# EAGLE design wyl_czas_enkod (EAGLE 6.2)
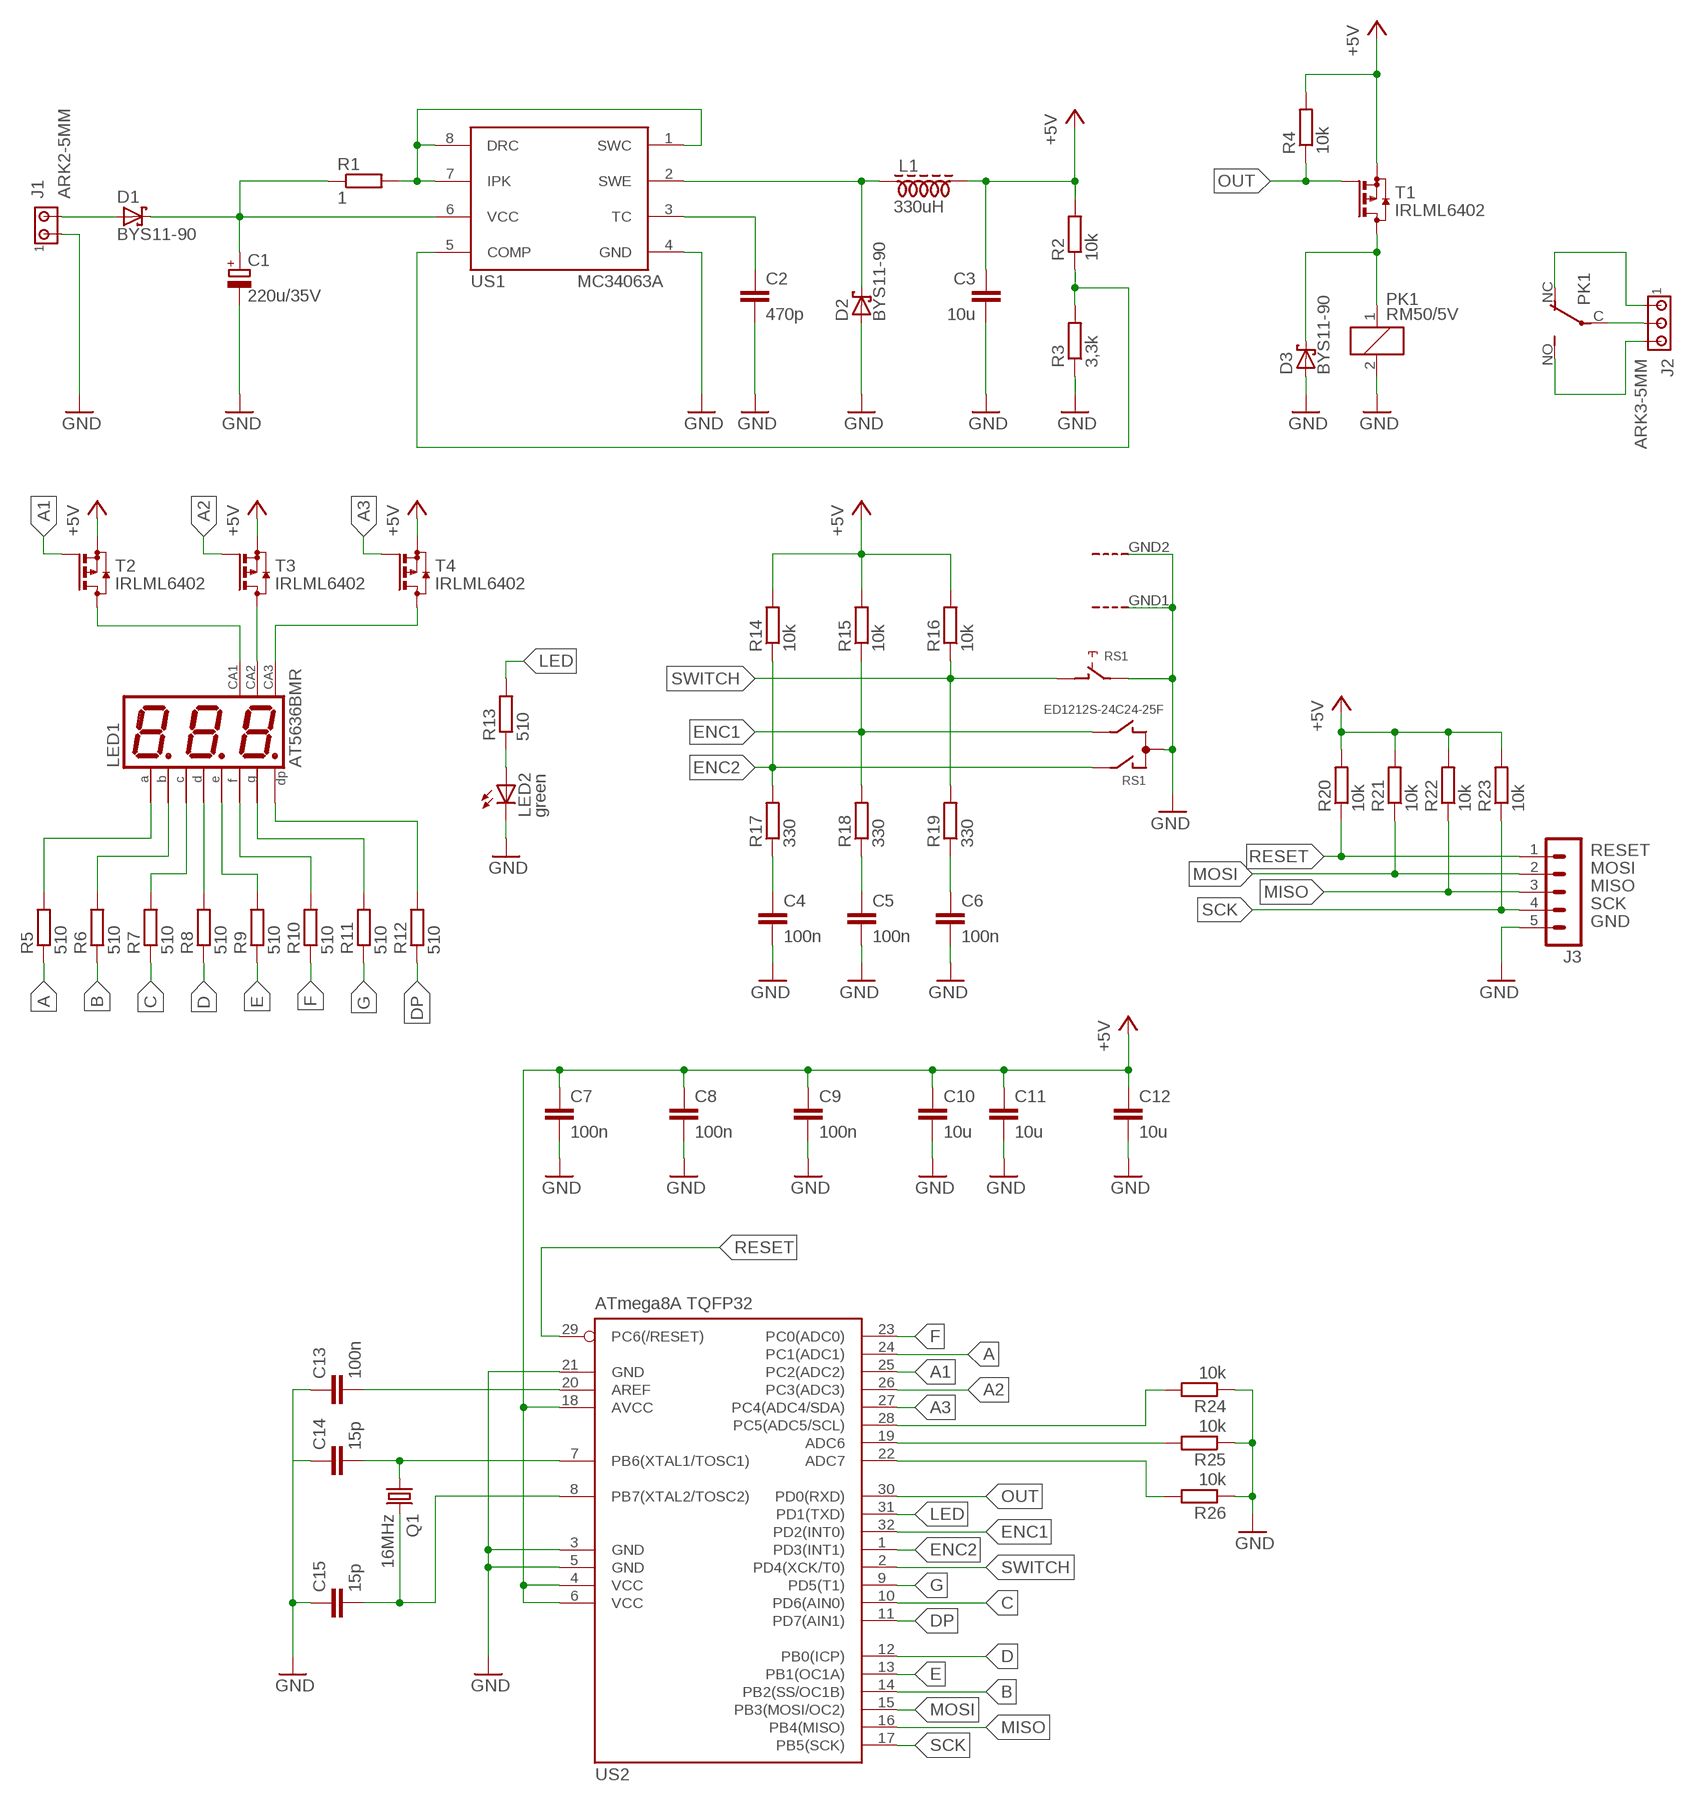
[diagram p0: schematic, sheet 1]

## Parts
C1  220u/35V  CPOL-EUE3.5-8  [E3,5-8]
C2  470p  C-EUC0805  [C0805]
C3  10u  C-EUC0805  [C0805]
C4  100n  C-EUC0805  [C0805]
C5  100n  C-EUC0805  [C0805]
C6  100n  C-EUC0805  [C0805]
C7  100n  C-EUC0805  [C0805]
C8  100n  C-EUC0805  [C0805]
C9  100n  C-EUC0805  [C0805]
C10  10u  C-EUC0805  [C0805]
C11  10u  C-EUC0805  [C0805]
C12  10u  C-EUC0805  [C0805]
C13  100n  C-EUC0805  [C0805]
C14  15p  C-EUC0805  [C0805]
C15  15p  C-EUC0805  [C0805]
D1  BYS11-90  SCHOTTKY-DIODESMD  [SMB]
D2  BYS11-90  SCHOTTKY-DIODESMD  [SMB]
D3  BYS11-90  SCHOTTKY-DIODESMD  [SMB]
J1  ARK2-5MM  [2PIN-5MM]
J2  ARK3-5MM  [3PIN-5MM]
J3  MA05-1  [MA05-1]
L1  330uH  DLAWIK-PION  [L_PION]
LED1  AT5636BMR  BC56-12SRWA  [BX56-12]
LED2  green  LED5MM  [LED5MM]
PK1  RM50/5V  PK_POJED-JQC-3FG  [PK_POJED_JQC-3FG]
Q1  16MHz  CRYSTALHC49UP  [HC49UP]
R1  1  R-EU_M0805  [M0805]
R2  10k  R-EU_M0805  [M0805]
R3  3,3k  R-EU_M0805  [M0805]
R4  10k  R-EU_M0805  [M0805]
R5  510  R-EU_M0805  [M0805]
R6  510  R-EU_M0805  [M0805]
R7  510  R-EU_M0805  [M0805]
R8  510  R-EU_M0805  [M0805]
R9  510  R-EU_M0805  [M0805]
R10  510  R-EU_M0805  [M0805]
R11  510  R-EU_M0805  [M0805]
R12  510  R-EU_M0805  [M0805]
R13  510  R-EU_M0805  [M0805]
R14  10k  R-EU_R0805  [R0805]
R15  10k  R-EU_R0805  [R0805]
R16  10k  R-EU_R0805  [R0805]
R17  330  R-EU_R0805  [R0805]
R18  330  R-EU_R0805  [R0805]
R19  330  R-EU_R0805  [R0805]
R20  10k  R-EU_R0805  [R0805]
R21  10k  R-EU_R0805  [R0805]
R22  10k  R-EU_R0805  [R0805]
R23  10k  R-EU_R0805  [R0805]
R24  10k  R-EU_R0805  [R0805]
R25  10k  R-EU_R0805  [R0805]
R26  10k  R-EU_R0805  [R0805]
RS1  ED1212S-24C24-25F  EC12E_SW  [ALPS_EC12E_SW]
T1  IRLML6402  BSS84  [SOT23]
T2  IRLML6402  BSS84  [SOT23]
T3  IRLML6402  BSS84  [SOT23]
T4  IRLML6402  BSS84  [SOT23]
US1  MC34063A  MC34063-SO8  [SO08]
US2  ATmega8A TQFP32  MEGA8-AI  [TQFP32-08]

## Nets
+5V: C3.1 C7.1 C8.1 C9.1 C10.1 C11.1 C12.1 L1.P$2 R2.2 R4.2 R14.2 R15.2 R16.2 R20.2 R21.2 R22.2 R23.2 T1.2(S) T2.2(S) T3.2(S) T4.2(S) US2.4(VCC) US2.6(VCC) US2.18(AVCC)
A: R5.1 US2.24(PC1(ADC1))
A1: T2.1(G) US2.25(PC2(ADC2))
A2: T3.1(G) US2.26(PC3(ADC3))
A3: T4.1(G) US2.27(PC4(ADC4/SDA))
B: R6.1 US2.14(PB2(SS/OC1B))
C: R7.1 US2.10(PD6(AIN0))
D: R8.1 US2.12(PB0(ICP))
DP: R12.1 US2.11(PD7(AIN1))
E: R9.1 US2.13(PB1(OC1A))
ENC1: R15.1 R18.2 RS1.B US2.32(PD2(INT0))
ENC2: R14.1 R17.2 RS1.A US2.1(PD3(INT1))
F: R10.1 US2.23(PC0(ADC0))
G: R11.1 US2.9(PD5(T1))
GND: C1.- C2.2 C3.2 C4.2 C5.2 C6.2 C7.2 C8.2 C9.2 C10.2 C11.2 C12.2 C13.1 C14.1 C15.1 D2.A D3.A J1.P$1 J3.5 LED2.K(C) PK1.2 R3.1 R24.1 R25.1 R26.1 RS1.C RS1.E RS1.GND1(G) RS1.GND2(G) US1.4(GND) US2.3(GND) US2.5(GND) US2.21(GND)
LED: R13.2 US2.31(PD1(TXD))
MISO: J3.3 R22.1 US2.16(PB4(MISO))
MOSI: J3.2 R21.1 US2.15(PB3(MOSI/OC2))
N$1: C6.1 R19.1
N$2: LED2.A R13.1
N$3: C15.2 Q1.2 US2.8(PB7(XTAL2/TOSC2))
N$4: C13.2 US2.20(AREF)
N$5: R25.2 US2.19(ADC6)
N$6: R24.2 US2.28(PC5(ADC5/SCL))
N$7: J2.P$1 PK1.NC
N$8: J2.P$3 PK1.NO
N$9: R2.1 R3.2 US1.5(COMP)
N$10: C14.2 Q1.1 US2.7(PB6(XTAL1/TOSC1))
N$11: LED1.9(CA) T3.3(D)
N$12: R26.2 US2.22(ADC7)
N$14: LED1.12(CA) T2.3(D)
N$15: LED1.8(CA) T4.3(D)
N$16: LED1.11(A) R5.2
N$17: LED1.7(B) R6.2
N$18: LED1.4(C) R7.2
N$19: LED1.2(D) R8.2
N$20: LED1.1(E) R9.2
N$21: LED1.10(F) R10.2
N$22: LED1.5(G) R11.2
N$23: LED1.3(DP) R12.2
N$31: D1.A J1.P$2
N$32: C1.+ D1.C R1.1 US1.6(VCC)
N$34: J2.P$2 PK1.C(COM)
N$35: C5.1 R18.1
N$36: C4.1 R17.1
N$37: R1.2 US1.1(SWC) US1.7(IPK) US1.8(DRC)
N$38: C2.1 US1.3(TC)
N$39: D2.C L1.P$1 US1.2(SWE)
N$40: D3.C PK1.1 T1.3(D)
OUT: R4.1 T1.1(G) US2.30(PD0(RXD))
RESET: J3.1 R20.1 US2.29(PC6(/RESET))
SCK: J3.4 R23.1 US2.17(PB5(SCK))
SWITCH: R16.1 R19.2 RS1.D US2.2(PD4(XCK/T0))

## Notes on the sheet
- RESET
- MOSI
- MISO
- SCK
- GND

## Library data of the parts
C1 = rcl:CPOL-EU: POLARIZED CAPACITOR, European symbol
C2-C15 = rcl:C-EU: CAPACITOR, European symbol
D1-D3 = diode:SCHOTTKY-DIODE: Schottky Diode
J1 = zlacza_futrzak:ARK2: ARK 2
J2 = zlacza_futrzak:ARK3: ARK 3 Raster 5mm i 3,5mm
J3 = zlacza_futrzak:MA05-1: PIN HEADER; OC_FARNELL: unknown; OC_NEWARK: unknown
L1 = inne_futrzak:DLAWIK
LED1 = display-kingbright:B?56-12*WA: 14.22mm (0.56INCH) THREE DIGIT NUMERIC DISPLAY Source: http://www.kingbright.com .. BA56-11EWA(Ver1189474895.pdf; OC_FARNELL: unknown; OC_NEWARK: unknown
LED2 = led:LED: LED
PK1 = inne_futrzak:PK_POJED
Q1 = crystal:CRYSTAL: CRYSTAL; OC_FARNELL: unknown; OC_NEWARK: unknown
R1-R26 = rcl:R-EU_: RESISTOR, European symbol
RS1 = switch-alps:EC12E_SW: ALPS rotary Encoder EC12E series with switch; MPN: EC12E2424407; OC_FARNELL: 1520813; OC_NEWARK: 74M1068
T1-T4 = transistor-small-signal:BSS84: P-CHANNEL MOS FET
US1 = scalaki_futrzak:MC34063
US2 = atmel:MEGA8: MICROCONTROLLER 8 Kbytes FLASH, 1 kbytes SRAM, 512 bytes EEPROM, USART, 6-channel 10 bit ADC, 2-channel 8 bit ADC Pin compatible with Atmega48, ATMega88, ATMega168 Source: avr.lbr; MPN: ATMEGA8-16AU; OC_FARNELL: 9171371; OC_NEWARK: 73M8863

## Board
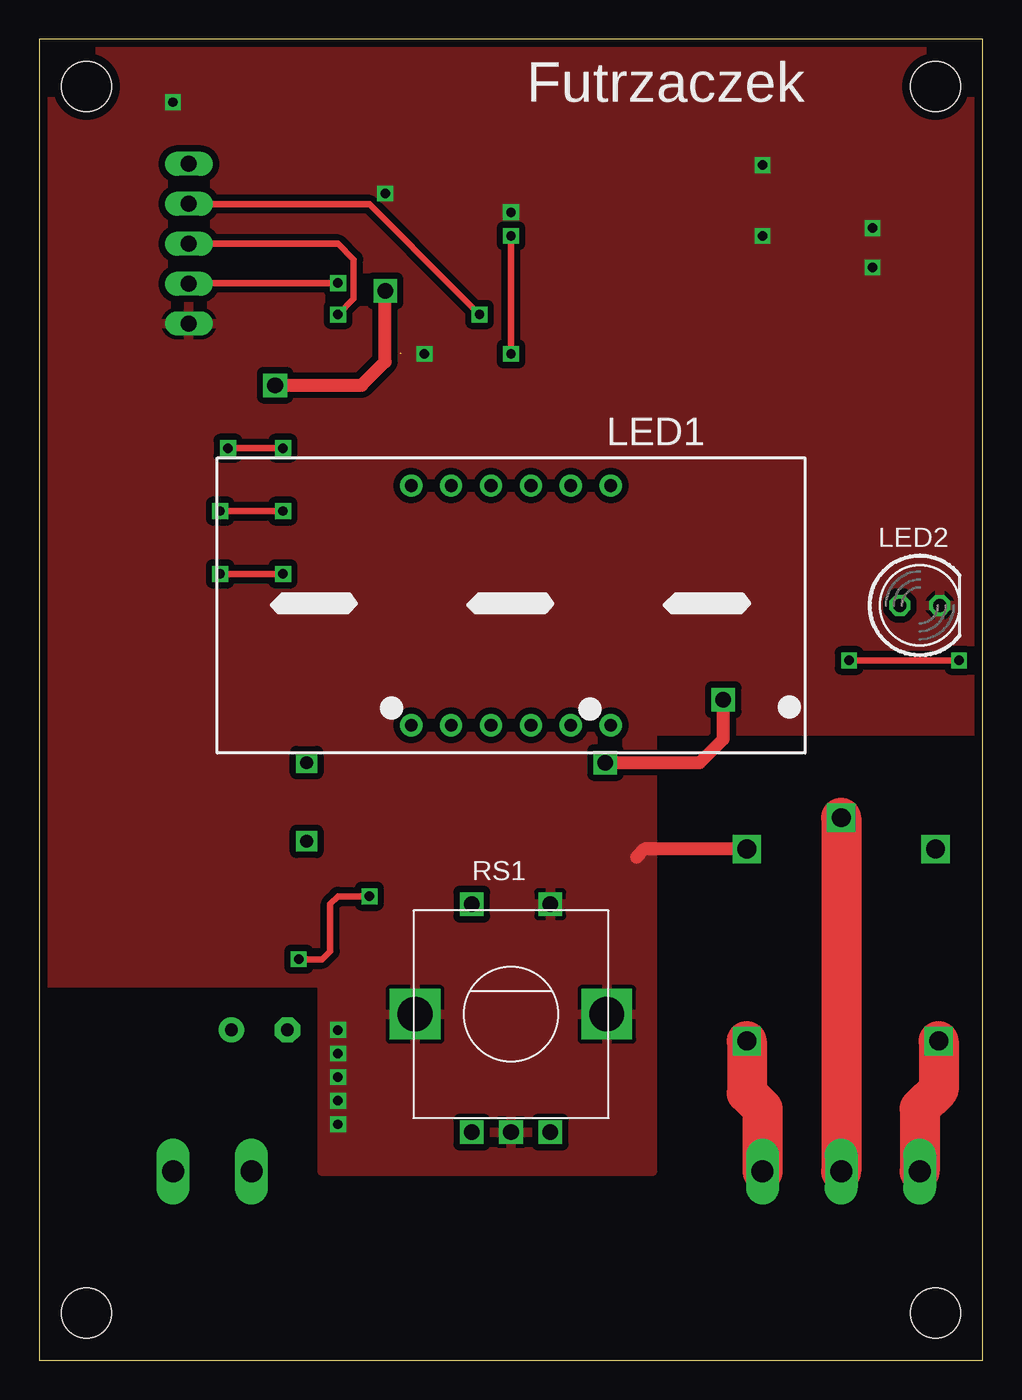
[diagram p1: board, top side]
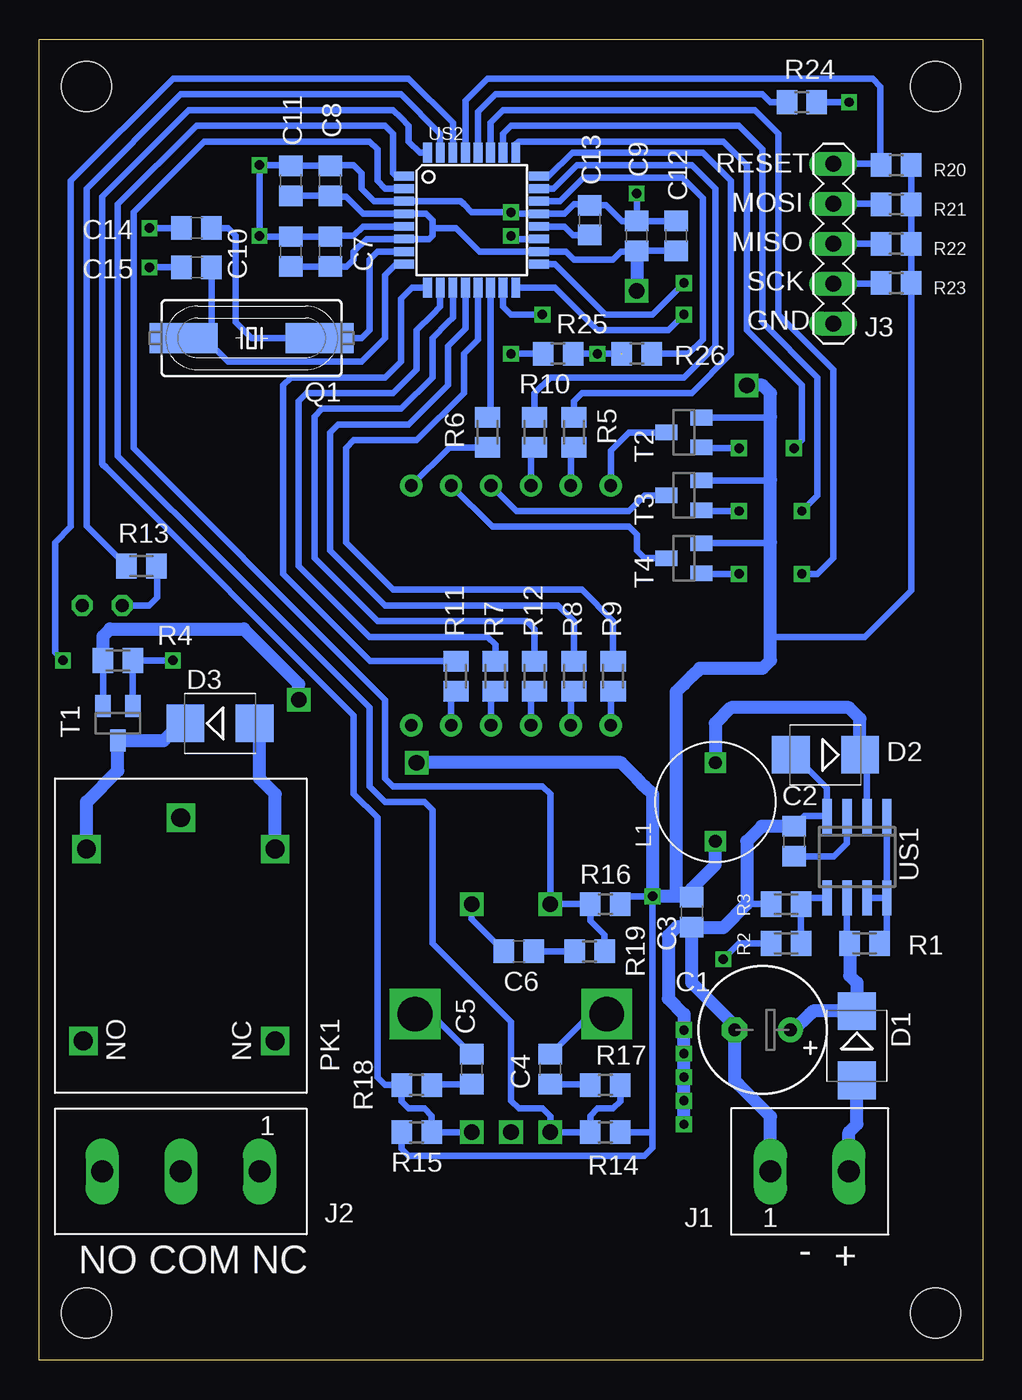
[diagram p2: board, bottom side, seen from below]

Size 60 x 84 mm. Coordinates in mm from the lower left corner, seen from the top.
Outline: 0,0 60,0 60,84 0,84 0,0
Copper layers (1*16): Top 0.035mm / dielectric 1.5mm / Bottom 0.035mm
Design rules: minimum track width 10mil, minimum drill 23mil, track to track 8mil, track to pad 8mil, pad to pad 8mil, via to via 8mil, smd to smd 8mil, copper to edge 20mil, drill to drill 8mil, minimum pad ring 10mil, minimum via ring 8mil, stop-mask expansion 4mil, vias tented up to drill 0mil, thermal gap 10mil
Holes 3.2 mm at 3,3 57,3 3,81 57,81

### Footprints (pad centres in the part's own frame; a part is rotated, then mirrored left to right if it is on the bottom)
E3,5-8 = drill 0.813 pad 1.6: + -1.778,0 | drill 0.813 pad 1.6 octagon: - 1.778,0
C0805 = smd 1.3 x 1.5: 1 -0.95,0; 2 0.95,0
SMB = smd 2.4 x 2.4: A 2.2,0; C -2.2,0
2PIN-5MM = drill 1.4 long: P$1 -2.5,0; P$2 2.5,0
3PIN-5MM = drill 1.4 long: P$1 -5,0; P$2 0,0; P$3 5,0
MA05-1 = drill 1.016 long: 1 -5.08,0; 2 -2.54,0; 3 0,0; 4 2.54,0; 5 5.08,0
L_PION = drill 0.8 square: P$1 -2.5,0; P$2 2.5,0
BX56-12 = drill 0.8 pad 1.422: 1 -6.35,-7.62; 2 -3.81,-7.62; 3 -1.27,-7.62; 4 1.27,-7.62; 5 3.81,-7.62; 6 6.35,-7.62; 7 6.35,7.62; 8 3.81,7.62; 9 1.27,7.62; 10 -1.27,7.62; 11 -3.81,7.62; 12 -6.35,7.62
LED5MM = drill 0.813 octagon: A -1.27,0; K 1.27,0
PK_POJED_JQC-3FG = drill 1.2 square: 1 5.5,6; 2 5.5,-6; C 7.5,0; NC -6.7,-6; NO -6.7,6.2
HC49UP = smd 4.318 x 1.93: 1 -4.318,0; 2 4.318,0
M0805 = smd 1.3 x 1.6: 1 -0.95,0; 2 0.95,0
R0805 = smd 1.3 x 1.5: 1 -0.95,0; 2 0.95,0
ALPS_EC12E_SW = drill 1 square: A -2.5,-7.5; B 2.5,-7.5; C 0,-7.5; D -2.5,7; E 2.5,7 | drill 2.2 square: GND1 -6.1,0; GND2 6.1,0
SOT23 = smd 1 x 1.4: 1 -0.95,-1.1; 2 0.95,-1.1; 3 0,1.1
SO08 = smd 0.6 x 2.2: 1 -1.905,-2.6; 2 -0.635,-2.6; 3 0.635,-2.6; 4 1.905,-2.6; 5 1.905,2.6; 6 0.635,2.6; 7 -0.635,2.6; 8 -1.905,2.6
TQFP32-08 = smd 1.27 x 0.559: 1 -4.293,2.8; 2 -4.293,2; 3 -4.293,1.2; 4 -4.293,0.4; 5 -4.293,-0.4; 6 -4.293,-1.2; 7 -4.293,-2; 8 -4.293,-2.8; 17 4.293,-2.8; 18 4.293,-2; 19 4.293,-1.2; 20 4.293,-0.4; 21 4.293,0.4; 22 4.293,1.2; 23 4.293,2; 24 4.293,2.8 | smd 0.559 x 1.27: 9 -2.8,-4.293; 10 -2,-4.293; 11 -1.2,-4.293; 12 -0.4,-4.293; 13 0.4,-4.293; 14 1.2,-4.293; 15 2,-4.293; 16 2.8,-4.293; 25 2.8,4.293; 26 2,4.293; 27 1.2,4.293; 28 0.4,4.293; 29 -0.4,4.293; 30 -1.2,4.293; 31 -2,4.293; 32 -2.8,4.293

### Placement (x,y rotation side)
C1  14,21 180 bottom
C2  12,33 90 bottom
C3  18.5,28.5 270 bottom
C4  27.5,18.5 90 bottom
C5  32.5,18.5 90 bottom
C6  29.5,26 180 bottom
C7  41.5,70.5 90 bottom
C8  41.5,75 90 bottom
C9  22,71.5 90 bottom
C10  44,70.5 90 bottom
C11  44,75 90 bottom
C12  19.5,71.5 90 bottom
C13  25,72.5 270 bottom
C14  50,72 0 bottom
C15  50,69.5 0 bottom
D1  8,20 270 bottom
D2  10,38.5 180 bottom
D3  48.5,40.5 0 bottom
J1  11,12 0 bottom
J2  51,12 180 bottom
J3  9.5,71 270 bottom
L1  17,35.5 270 bottom
LED1  30,48 0 top
LED2  56,48 0 top
PK1  51,27 90 bottom
Q1  46.5,65 180 bottom
R1  7.5,26.5 0 bottom
R2  12.5,26.5 180 bottom
R3  12.5,29 0 bottom
R4  55,44.5 180 bottom
R5  26,59 270 bottom
R6  31.5,59 270 bottom
R7  31,43.5 270 bottom
R8  26,43.5 270 bottom
R9  23.5,43.5 270 bottom
R10  28.5,59 270 bottom
R11  33.5,43.5 270 bottom
R12  28.5,43.5 270 bottom
R13  53.5,50.5 180 bottom
R14  24,14.5 0 bottom
R15  36,14.5 180 bottom
R16  24,29 0 bottom
R17  24,17.5 0 bottom
R18  36,17.5 180 bottom
R19  25,26 0 bottom
R20  5.5,76 0 bottom
R21  5.5,73.5 0 bottom
R22  5.5,71 0 bottom
R23  5.5,68.5 0 bottom
R24  11.5,80 180 bottom
R25  27,64 180 bottom
R26  22,64 0 bottom
RS1  30,22 0 top
T1  55,40.5 180 bottom
T2  19,59 90 bottom
T3  19,55 90 bottom
T4  19,51 90 bottom
US1  8,32 180 bottom
US2  32.5,72.5 0 bottom

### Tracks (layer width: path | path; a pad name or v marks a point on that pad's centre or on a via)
+5V  (via drill 0.6, 1)
  Top 0.406: v16.5,25.5 18,25.5 18.5,26 18.5,29 19,29.5 v21,29.5
  Top 0.813: v36,38 42,38 43.5,39.5 v43.5,42 | v15,62 19,62 20.5,62 22,63.5 v22,68
  Bottom 0.406: R2.2 15.5,26.5 16,26 v16.5,25.5 | 18.55,29.5 C3.1 | R15.2 36.95,13.45 36.5,13 21.5,13 21,13.5 21,14.5 | 21,14.5 v21,29.5 22.5,29.5 23,29 R16.2 | R14.2 21,14.5 | R4.2 T1.2 | T4.2 13.55,51.95 13.5,52 | T2.2 13.55,59.95 13.5,60 | T3.2 13.55,55.95 13.5,56 | C12.1 C9.1 22.05,70.5 23,70.5 23.5,70 26,70 26.5,70.5 US2.18 30.5,70.5 32,70.5 33.5,72 35,72 | C11.1 C8.1 41.45,74 40.5,74 39.4,72.9 US2.4 35.4,72.9 35,72.5 35,72 | C10.1 C7.1 40.45,69.55 40,70 40,70.5 39.2,71.3 US2.6 35.2,71.3 35,71.5 35,72 | R20.2 R21.2 R22.2 R23.2 4.55,48.95 7.5,46 13.5,46
  Bottom 0.813: C3.1 18.5,30 17,31.5 L1.P$2 | R4.2 55.95,46.05 55.5,46.5 47,46.5 43.5,43 v43.5,42 | 18.55,29.5 19.5,29.5 | 19.5,29.5 v21,29.5 21,36 21.5,36.5 22,37 23,38 v36,38 | 19.5,29.5 19.5,42.5 19,43 18.5,43.5 18,44 14,44 13.5,44.5 13.5,46 13.5,52 13.5,56 13.5,60 13.5,61.5 14,62 v15,62 | C9.1 v22,68
A
  Bottom 0.406: R5.1 26,61 25.5,61.5 24.45,61.5 18.5,61.5 16,64 16,75 16.5,75.5 17.5,76.5 17.8,76.8 26.1,76.8 27.6,75.3 US2.24
A1  (via drill 0.6)
  Top 0.406: v12,58 v15.5,58
  Bottom 0.406: US2.25 29.7,77.3 29.5,77.5 16.5,77.5 15.5,76.5 15,76 15,65.5 11.5,62 11.5,58.5 v12,58 | v15.5,58 17.85,58 T2.1
A2  (via drill 0.6)
  Top 0.406: v11.5,54 v15.5,54
  Bottom 0.406: US2.26 30.5,78 30,78.5 15.5,78.5 14.5,77.5 14,77 14,66 10.5,62.5 10.5,55 v11.5,54 | v15.5,54 17.85,54 T3.1
A3  (via drill 0.6)
  Top 0.406: v11.5,50 v15.5,50
  Bottom 0.406: US2.27 31.3,78.7 30.5,79.5 14.5,79.5 13.5,78.5 13,78 13,66.5 9.5,63 9.5,51 10.5,50 v11.5,50 | v15.5,50 17.85,50 T4.1
B
  Bottom 0.406: US2.14 31.3,60.15 R6.1
C
  Bottom 0.406: R7.1 31,45.5 31.5,46 39,46 43.5,50.5 43.5,61 43,61.5 37.5,61.5 36,63 36,65.5 35,66.5 34.5,67 US2.10
D
  Bottom 0.406: R8.1 26,47 27,48 38,48 41.5,51.5 41.5,59 41,59.5 36.5,59.5 34,62 34,64.5 33,65.5 32.9,65.6 US2.12
DP
  Bottom 0.406: R12.1 28.5,46.5 29,47 38.5,47 42.5,51 42.5,60 42,60.5 37,60.5 35,62.5 35,65 34,66 33.7,66.3 US2.11
E
  Bottom 0.406: R9.1 23.5,47 25.5,49 37.5,49 40.5,52 40.5,58 40,58.5 36,58.5 33,61.5 33,64 32.5,64.5 32.1,64.9 US2.13
ENC1
  Bottom 0.406: US2.32 35.79,76.79 36.5,77.5 36.5,78.5 37,79 37.5,79.5 50.5,79.5 56,74 56,57 | 56,57 55.75,56.75 | 55.75,56.75 40,41 40,36 38.5,34.5 38.5,18 38,17.5 R18.2 36.95,16.45 36.5,16 35.5,16 35.05,15.55 R15.1 RS1.B | 56,57 55.75,56.75
ENC2
  Bottom 0.406: R17.2 23.05,16.45 23.5,16 24.5,16 24.95,15.55 R14.1 RS1.A 27.5,15.5 28,16 28.5,16 29.5,16 30,16.5 30,21.5 35,26.5 35,35 35.5,35.5 38,35.5 39,36.5 39,41.5 41,43.5 48,50.5 55,57.5 55,73.5 50,78.5 38,78.5 37.5,78 37.5,75.5 37.3,75.3 US2.1
F
  Bottom 0.406: R10.1 28.5,61.5 27.5,62.5 19,62.5 17,64.5 17,74.5 18,75.5 18.5,76 25.8,76 25.9,75.9 27.3,74.5 US2.23
G
  Bottom 0.406: R11.1 38.95,44.45 44.5,50 44.5,62 44,62.5 38,62.5 37,63.5 37,67.5 36.5,68 36.29,68.21 US2.9
GND  (via drill 0.6)  (1 unrouted)
  Top 0.813: PK1.2 38.5,32.5 38,32
  Bottom 0.406: C2.2 11.35,34.6 US1.4 9.9,36.41 10,36.5 12,38.5 D2.A | R3.1 15,29 | RS1.GND1 24.95,22 C4.2 | RS1.GND2 35.05,22 C5.2 | C14.1 v53,72 | v53,69.5 C15.1 | C9.2 C12.2 | 41.45,76 C8.2 | C11.2 43.5,75.95 | 43.5,75.95 C8.2 | US2.5 39.4,72.1 40,71.5 41.45,71.5 C7.2 C10.2 45.95,71.45 v46,71.5 v46,76 43.55,76 43.5,75.95 | 41.45,76 40,76 39.5,75.5 39.5,74.5 38.7,73.7 38.2,73.7 US2.3 33.2,73.7 33,73.5 32.5,73 v30,73 29.9,72.9 US2.21 26.6,72.9 26,73.5 25.05,73.5 C13.1 23.95,73.45 23.5,73 22.95,72.45 C9.2 | 41.45,76 C8.2 | RS1.E 32.5,28.05 C6.2 | R24.1 v8.5,80 | R25.1 v24.5,64 23,64 | C9.2 v22,74.2
  Bottom 0.813: C2.2 14.05,33.95 15,33 15,29 16.5,27.5 18.45,27.5 C3.2 19,27.55 | PK1.2 45,36 46,37 46,40.2 D3.A | J1.P$1 13.5,15.5 15.5,17.5 15.78,17.78 C1.- 15.78,21.28 18.5,24 18.5,27.05 19,27.55 | 19,27.55 19.45,27.55 20,27 20,23 19,22 v19,21 v19,19.5 v19,18 v19,16.5 v19,15
  pour Top (isolate 0.406): 0,24 18,24 18,12 39,12 39,40 60,40 60,84 0,84
LED
  Bottom 0.406: US2.31 34.5,78 37,80.5 51,80.5 57,74.5 57,53.05 R13.2
MISO  (via drill 0.6)
  Top 0.406: v19,66.5 20,67.5 20,70 19,71 J3.3
  Bottom 0.406: J3.3 R22.1 | US2.16 27.21,68.21 24.5,65.5 20,65.5 v19,66.5
MOSI  (via drill 0.6)
  Top 0.406: v28,66.5 26.5,68 21,73.5 9.54,73.5 J3.2
  Bottom 0.406: J3.2 6.49,73.54 R21.1 | US2.15 30.5,67 30,66.5 v28,66.5
N$1
  Bottom 0.406: C6.1 R19.1
N$2
  Bottom 0.406: LED2.A 53,48 52.5,48.5 52.5,50.45 R13.1
N$3
  Bottom 0.406: C15.2 49.05,65.45 49.5,65 | 49.5,65 Q1.2 | US2.8 37.3,69.7 38,69 38,65 39.5,63.5 48,63.5 49.5,65
N$4
  Bottom 0.406: US2.20 26.6,72.1 26.5,72 26.05,71.55 C13.2
N$5  (via drill 0.6)
  Top 0.406: v30,64 v30,71.5
  Bottom 0.406: R25.2 v30,64 | US2.19 29.8,71.3 v30,71.5
N$6
  Bottom 0.406: US2.28 32.1,79.4 31,80.5 14,80.5 13.5,80 R24.2
N$7
  Top 2.54: PK1.NC 45,17 46,16 J2.P$1
N$8
  Top 2.54: PK1.NO 57.2,17.2 56,16 J2.P$3
N$9
  Bottom 0.406: US1.5 11.15,29.4 R3.2 R2.1
N$10
  Bottom 0.406: US2.7 38.5,70.5 39,70 39,68 39,65.5 39.5,65 Q1.1 | Q1.1 43,65 | 43,65 Q1.1 | C14.2 48,72 47.5,71.5 47.5,66 46.5,65 43,65
N$11
  Bottom 0.406: T3.3 21.5,55 22,54.5 22.5,54 29.65,54 LED1.9
N$12
  Bottom 0.406: R26.2 18.7,64 17.8,64.9 17.8,73.9 19.1,75.2 25.4,75.2 26.9,73.7 US2.22
N$14
  Bottom 0.406: LED1.12 23.65,57.85 22.5,59 T2.3
N$15
  Bottom 0.406: T4.3 21.5,51 22,51.5 22,52.5 22.5,53 31.19,53 LED1.8
N$16
  Bottom 0.406: LED1.11 26.19,57.86 R5.2
N$17
  Bottom 0.406: R6.2 33.92,58.05 LED1.7
N$18
  Bottom 0.406: LED1.4 31.27,42.28 R7.2
N$19
  Bottom 0.406: LED1.2 26.19,42.36 R8.2
N$20
  Bottom 0.406: LED1.1 23.65,42.4 R9.2
N$21
  Bottom 0.406: LED1.10 28.73,57.82 R10.2
N$22
  Bottom 0.406: LED1.5 33.81,42.24 R11.2
N$23
  Bottom 0.406: LED1.3 28.73,42.32 R12.2
N$31
  Bottom 0.813: J1.P$2 8.5,14.5 8,15 8,17 D1.A
N$32
  Bottom 0.406: US1.6 8.63,26.68 R1.1
  Bottom 0.813: C1.+ 12,21 11,22 10.8,22.2 D1.C 8,24 8.45,24.45 R1.1
N$34
  Top 2.54: PK1.C J2.P$2
N$35
  Bottom 0.406: C5.1 35,17.55 R18.1
N$36
  Bottom 0.406: C4.1 25,17.55 R17.1
N$37
  Bottom 0.406: US1.8 6.09,26.95 R1.2 | US1.7 US1.8 | US1.1 US1.8
N$38
  Bottom 0.406: C2.1 9.45,32.05 9,32.5 8.63,32.87 US1.3
N$39
  Bottom 0.406: US1.2 7.37,38.06 D2.C
  Bottom 0.813: D2.C 7.8,40.8 8.5,41.5 16,41.5 17,40.5 L1.P$1
N$40
  Bottom 0.813: PK1.1 57,35.5 55,37.5 T1.3 52.1,39.4 52,39.5 51,40.5 D3.C
OUT  (via drill 0.6)
  Top 0.406: v58.5,44.5 v51.5,44.5
  Bottom 0.406: T1.1 R4.1 v51.5,44.5 | US2.30 33.7,78.7 36.5,81.5 51.5,81.5 58,75 58,53 59,52 59,45 v58.5,44.5
RESET
  Bottom 0.406: J3.1 6.53,76.08 R20.1 6.5,76.05 6.5,81 7,81.5 10.5,81.5 31.5,81.5 32.9,80.1 US2.29
SCK  (via drill 0.6)
  Top 0.406: v19,68.5 9.54,68.5 J3.4
  Bottom 0.406: J3.4 6.49,68.46 R23.1 | US2.17 27.2,69.7 24,66.5 21,66.5 v19,68.5
SWITCH
  Bottom 0.406: US2.2 38,74.5 38.5,75 38.5,77 39,77.5 49.5,77.5 54,73 54,58 40,44 38,42 38,37 37.5,36.5 28,36.5 27.5,36 RS1.D R16.1 24.95,27.95 24.5,27.5 24.05,27.05 R19.2

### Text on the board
tPlace: Futrzaczek
bPlace: RESET | MOSI | MISO | SCK | GND | + - | NO COM NC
